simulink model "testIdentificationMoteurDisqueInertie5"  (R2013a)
settings: Solver=ode45  StartTime=0  StopTime=1  FixedStep=1e-3  MaxStep=SimParam.Control.Te  RelTol=1e-3  AbsTol=1e-4
PreLoadFcn:
  | warning('off','sm:sli:setup:compile:LocalSolverNotSupported')
model workspace (MAT data in the model file):
  handle : class17 (value not decoded)
  handle : class17 (value not decoded)
undefined symbols (not defined in the file or in its folder): SimParam

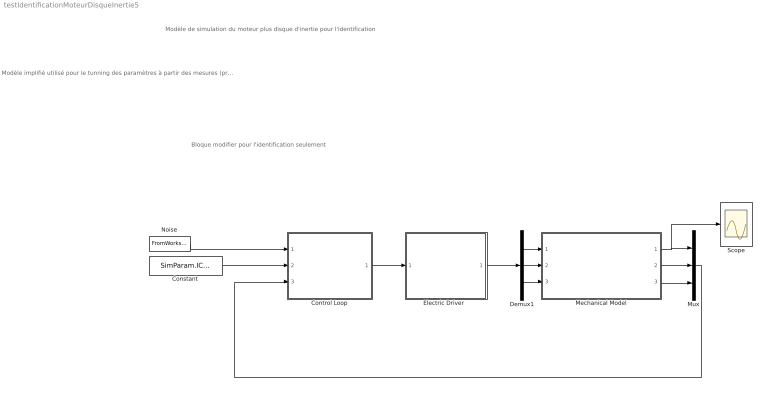
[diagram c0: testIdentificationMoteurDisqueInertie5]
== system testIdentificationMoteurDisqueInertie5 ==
  note: Bloque modifier pour l'identification seulement
  note: Modèle de simulation du moteur plus disque d'inertie pour l'identification
  note: Modèle implifié utilisé pour le tunning des paramètres à partir des mesures (prbs) effectuée sur le robot (Idem testIdentificationMoteur mais avec un élèment flexible dans le moteur) - Régulateur PID simple avec quantification codeur - Alimentation éléctrique modélisée par une fonction de transfert d'ordre deux avec delais (delais du contrôle) - Méchanique comprennant uniquement un modèle du moteur (inertie + frottement + 1ddl flexible en torsion) + frottement sec - Signaux d'exitation comprennant un bruit blanc et un signal cyclique (PRBS)
  Constant : Constant  Value=SimParam.IC.Alpha
  Control Loop : Subsystem  Variant=on
  Demux1 : Demux  Outputs=3
  "Electric Driver  " : Subsystem  Variant=on
  Mechanical Model : ModelReference  ModelNameDialog=ArmOnly_sm2_v2.slx  ModelReferenceVersion=1.266  CopyOfModelName=ArmOnly_sm2_v2.slx  DefaultDataLogging=on
  Mux : Mux  Inputs=3
  Noise : FromWorkspace  VariableName=SimIn  SampleTime=SimParam.Control.Te  Interpolate=off  OutputAfterFinalValue=Holding final value
  Scope : Scope
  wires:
  Constant/1 -> Control Loop/2(Alpha_c)
  Control Loop/1(U) -> "Electric Driver  "/1(U)
  Mux/1 -> Control Loop/3(Alpha)
  "Electric Driver  "/1(Torque) -> Demux1/1
  Noise/1 -> Control Loop/1(Noise)
  Demux1/1 -> Mechanical Model/1
  Demux1/2 -> Mechanical Model/2
  Demux1/3 -> Mechanical Model/3
  Mechanical Model/3 -> Mux/3
  Mechanical Model/2 -> Mux/2
  Mechanical Model/1 -> Scope/1, Mux/1

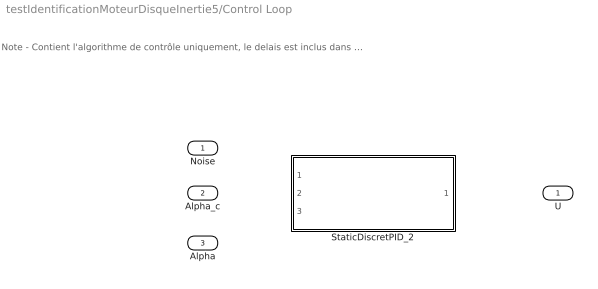
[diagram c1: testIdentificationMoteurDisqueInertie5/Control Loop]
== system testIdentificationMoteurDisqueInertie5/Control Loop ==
  note: Note - Contient l'algorithme de contrôle uniquement, le delais est inclus dans le bloque 'Electric Drive'
  Noise : Inport
  Alpha_c : Inport  Port=2
  Alpha : Inport  Port=3
  StaticDiscretPID_2 : Subsystem  VariantControl=controlVarDefault
  U : Outport

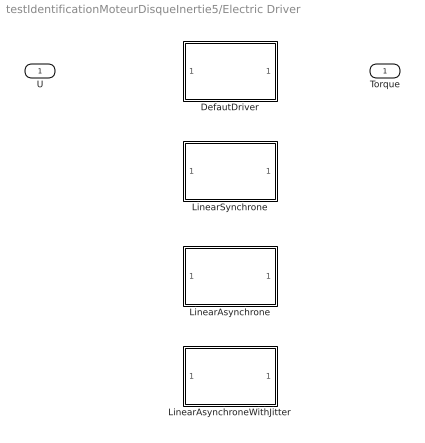
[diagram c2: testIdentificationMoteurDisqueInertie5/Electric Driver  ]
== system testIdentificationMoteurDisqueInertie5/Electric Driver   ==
  U : Inport
  DefautDriver : Subsystem  VariantControl=driverVarDefault
  LinearAsynchrone : Subsystem  VariantControl=driverVarLinearAsynchrone
  LinearAsynchroneWithJitter : Subsystem  VariantControl=driverVarLinearAsynchroneWithJitter
  LinearSynchrone : Subsystem  VariantControl=driverVarLinearSynchrone
  Torque : Outport

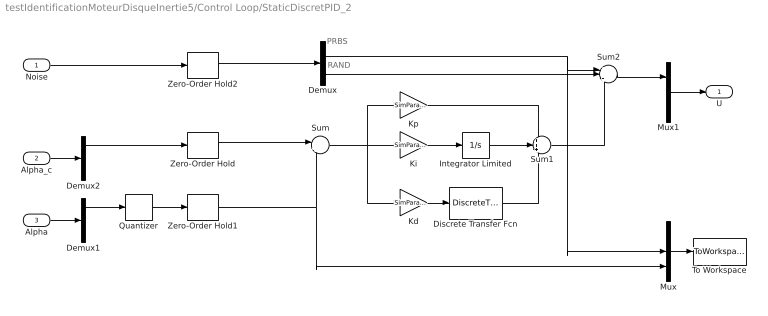
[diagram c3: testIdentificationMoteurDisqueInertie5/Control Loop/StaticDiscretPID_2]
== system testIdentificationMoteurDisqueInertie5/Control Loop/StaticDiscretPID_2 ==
  note: RAND
  note: PRBS
  Noise : Inport
  Alpha_c : Inport  Port=2
  Alpha : Inport  Port=3
  Demux : Demux  Outputs=2
  Demux1 : Demux  Outputs=3
  Demux2 : Demux  Outputs=3
  Discrete Transfer Fcn : DiscreteTransferFcn  Numerator=[1 0 -1]  Denominator=[2 0 0]
  Integrator Limited : Integrator  LimitOutput=on  UpperSaturationLimit=1  LowerSaturationLimit=-1
  Kd : Gain  Gain=SimParam.Control.Kd/SimParam.Control.Te
  Ki : Gain  Gain=SimParam.Control.Ki*SimParam.Control.Te
  Kp : Gain  Gain=SimParam.Control.Kp
  Mux : Mux  Inputs=3
  Mux1 : Mux  Inputs=3
  Quantizer : Quantizer  QuantizationInterval=2*pi/(4500*4*25)
  Sum : Sum  Inputs=|+-
  Sum1 : Sum  Inputs=+++
  Sum2 : Sum  Inputs=+++
  To Workspace : ToWorkspace  VariableName=simout  SampleTime=SimParam.Control.Te  SaveFormat=Structure With Time
  Zero-Order Hold : ZeroOrderHold  SampleTime=SimParam.Control.Te
  Zero-Order Hold1 : ZeroOrderHold  SampleTime=SimParam.Control.Te
  Zero-Order Hold2 : ZeroOrderHold  SampleTime=SimParam.Control.Te
  U : Outport
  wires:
  Kd/1 -> Discrete Transfer Fcn/1
  Mux/1 -> To Workspace/1
  Zero-Order Hold/1 -> Sum/1
  Quantizer/1 -> Zero-Order Hold1/1
  Noise/1 -> Zero-Order Hold2/1
  Discrete Transfer Fcn/1 -> Sum1/3
  Kp/1 -> Sum1/1
  Sum1/1 -> Sum2/3
  Demux/1 -> Mux/2, Sum2/1
  Ki/1 -> Integrator Limited/1
  Integrator Limited/1 -> Sum1/2
  Sum/1 -> Ki/1, Kp/1, Kd/1
  Zero-Order Hold1/1 -> Mux/3, Sum/2
  Demux/2 -> Sum2/2
  Zero-Order Hold2/1 -> Demux/1
  Demux1/1 -> Quantizer/1
  Alpha/1 -> Demux1/1
  Demux2/1 -> Zero-Order Hold/1
  Alpha_c/1 -> Demux2/1
  Mux1/1 -> U/1
  Sum2/1 -> Mux1/1

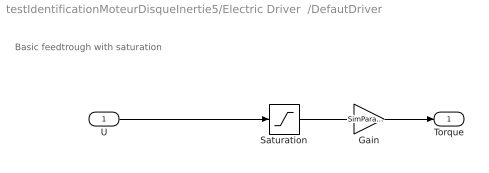
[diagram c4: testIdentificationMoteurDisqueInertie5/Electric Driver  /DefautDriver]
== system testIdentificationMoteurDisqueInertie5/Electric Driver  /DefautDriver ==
  note: Basic feedtrough with saturation
  U : Inport
  Gain : Gain  Gain=SimParam.Driver.GRelScale
  Saturation : Saturate  UpperLimit=SimParam.Driver.Sat  LowerLimit=-SimParam.Driver.Sat
  Torque : Outport
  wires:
  U/1 -> Saturation/1
  Saturation/1 -> Gain/1
  Gain/1 -> Torque/1

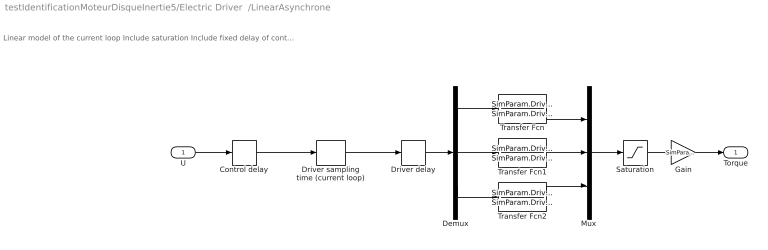
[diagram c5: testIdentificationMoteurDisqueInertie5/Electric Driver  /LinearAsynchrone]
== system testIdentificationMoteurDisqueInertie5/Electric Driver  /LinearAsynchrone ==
  note: Linear model of the current loop Include saturation Include fixed delay of control and driver and sampling time
  U : Inport
  Control delay : TransportDelay  DelayTime=SimParam.Driver.tau1
  Demux : Demux  Outputs=3
  Driver delay : TransportDelay  DelayTime=SimParam.Driver.tau1
  Driver sampling time (current loop) : ZeroOrderHold  SampleTime=SimParam.Driver.Te
  Gain : Gain  Gain=SimParam.Driver.GRelScale
  Mux : Mux  Inputs=3
  Saturation : Saturate  UpperLimit=SimParam.Driver.Sat  LowerLimit=-SimParam.Driver.Sat
  Transfer Fcn : TransferFcn  Numerator=SimParam.Driver.TfNum  Denominator=SimParam.Driver.TfDen
  Transfer Fcn1 : TransferFcn  Numerator=SimParam.Driver.TfNum  Denominator=SimParam.Driver.TfDen
  Transfer Fcn2 : TransferFcn  Numerator=SimParam.Driver.TfNum  Denominator=SimParam.Driver.TfDen
  Torque : Outport
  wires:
  U/1 -> Control delay/1
  Demux/1 -> Transfer Fcn/1
  Transfer Fcn/1 -> Mux/1
  Demux/3 -> Transfer Fcn2/1
  Transfer Fcn2/1 -> Mux/3
  Transfer Fcn1/1 -> Mux/2
  Demux/2 -> Transfer Fcn1/1
  Mux/1 -> Saturation/1
  Driver delay/1 -> Demux/1
  Control delay/1 -> Driver sampling time (current loop)/1
  Driver sampling time (current loop)/1 -> Driver delay/1
  Saturation/1 -> Gain/1
  Gain/1 -> Torque/1

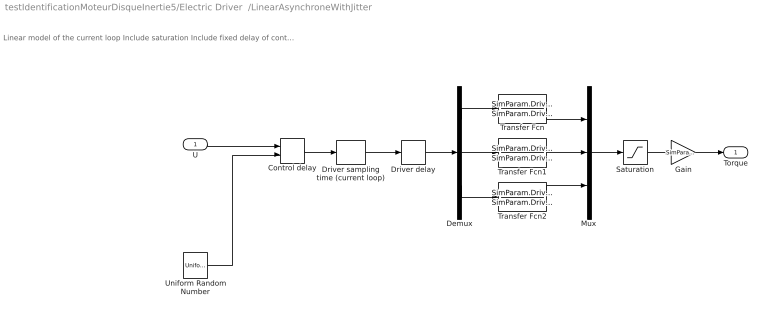
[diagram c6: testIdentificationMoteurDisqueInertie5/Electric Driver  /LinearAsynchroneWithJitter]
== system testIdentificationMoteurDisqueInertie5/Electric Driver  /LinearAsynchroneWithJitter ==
  note: Linear model of the current loop Include saturation Include fixed delay of control and driver and sampling time
  U : Inport
  Control delay : VariableTransportDelay  VariableDelayType=Variable transport delay  MaximumDelay=SimParam.Driver.tau1*2
  Demux : Demux  Outputs=3
  Driver delay : TransportDelay  DelayTime=SimParam.Driver.tau2
  Driver sampling time (current loop) : ZeroOrderHold  SampleTime=SimParam.Driver.Te
  Gain : Gain  Gain=SimParam.Driver.GRelScale
  Mux : Mux  Inputs=3
  Saturation : Saturate  UpperLimit=SimParam.Driver.Sat  LowerLimit=-SimParam.Driver.Sat
  Transfer Fcn : TransferFcn  Numerator=SimParam.Driver.TfNum  Denominator=SimParam.Driver.TfDen
  Transfer Fcn1 : TransferFcn  Numerator=SimParam.Driver.TfNum  Denominator=SimParam.Driver.TfDen
  Transfer Fcn2 : TransferFcn  Numerator=SimParam.Driver.TfNum  Denominator=SimParam.Driver.TfDen
  Uniform Random Number : UniformRandomNumber  Minimum=SimParam.Driver.tau1*0.99  Maximum=SimParam.Driver.tau1*1.01  SampleTime=SimParam.Control.Te
  Torque : Outport
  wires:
  U/1 -> Control delay/1
  Demux/1 -> Transfer Fcn/1
  Transfer Fcn/1 -> Mux/1
  Demux/3 -> Transfer Fcn2/1
  Transfer Fcn2/1 -> Mux/3
  Transfer Fcn1/1 -> Mux/2
  Demux/2 -> Transfer Fcn1/1
  Mux/1 -> Saturation/1
  Driver delay/1 -> Demux/1
  Control delay/1 -> Driver sampling time (current loop)/1
  Driver sampling time (current loop)/1 -> Driver delay/1
  Saturation/1 -> Gain/1
  Gain/1 -> Torque/1
  Uniform Random Number/1 -> Control delay/2

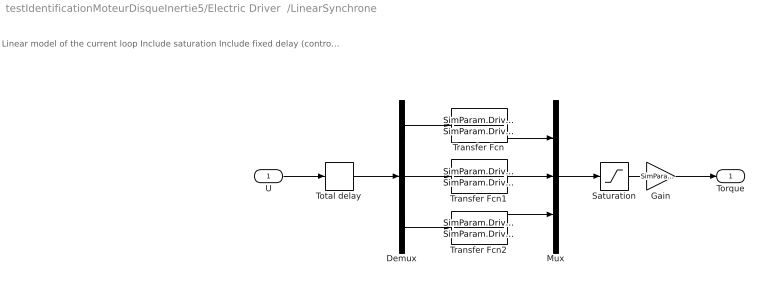
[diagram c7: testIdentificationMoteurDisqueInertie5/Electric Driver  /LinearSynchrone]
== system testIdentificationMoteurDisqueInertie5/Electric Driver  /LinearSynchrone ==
  note: Linear model of the current loop Include saturation Include fixed delay (control delay + driver delay + 0.5*driver sample periode if assynchonous)
  U : Inport
  Demux : Demux  Outputs=3
  Gain : Gain  Gain=SimParam.Driver.GRelScale
  Mux : Mux  Inputs=3
  Saturation : Saturate  UpperLimit=SimParam.Driver.Sat  LowerLimit=-SimParam.Driver.Sat
  Total delay : TransportDelay  DelayTime=SimParam.Driver.tau
  Transfer Fcn : TransferFcn  Numerator=SimParam.Driver.TfNum  Denominator=SimParam.Driver.TfDen
  Transfer Fcn1 : TransferFcn  Numerator=SimParam.Driver.TfNum  Denominator=SimParam.Driver.TfDen
  Transfer Fcn2 : TransferFcn  Numerator=SimParam.Driver.TfNum  Denominator=SimParam.Driver.TfDen
  Torque : Outport
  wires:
  U/1 -> Total delay/1
  Total delay/1 -> Demux/1
  Demux/1 -> Transfer Fcn/1
  Transfer Fcn/1 -> Mux/1
  Demux/3 -> Transfer Fcn2/1
  Transfer Fcn2/1 -> Mux/3
  Transfer Fcn1/1 -> Mux/2
  Demux/2 -> Transfer Fcn1/1
  Mux/1 -> Saturation/1
  Saturation/1 -> Gain/1
  Gain/1 -> Torque/1
